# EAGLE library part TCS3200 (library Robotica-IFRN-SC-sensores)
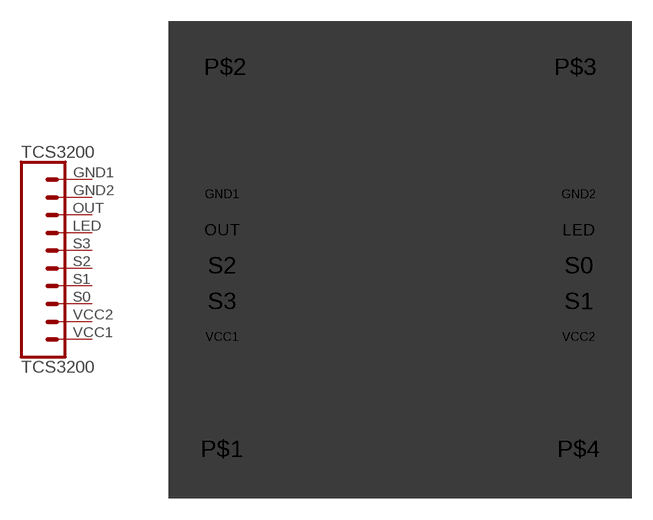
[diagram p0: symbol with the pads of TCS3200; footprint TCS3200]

Designator prefix TCS3200

## TCS3200  [TCS3200]
GND1  GND1  pas
GND2  GND2  pas
LED  LED  pas
OUT  OUT  pas
S0  S0  pas
S1  S1  pas
S2  S2  pas
S3  S3  pas
VCC1  VCC1  pas
VCC2  VCC2  pas

## Footprint TCS3200 (pad centres in mm)
drill 1.118 pad 1.88 long: GND1 -12.69,3.91; GND2 12.71,3.91; LED 12.71,1.37; OUT -12.69,1.37; S0 12.71,-1.17; S1 12.71,-3.71; S2 -12.69,-1.17; S3 -12.69,-3.71; VCC1 -12.69,-6.25; VCC2 12.71,-6.25
drill 2.8: P$1 -12.7,-14.24; P$2 -12.47,12.97; P$3 12.47,12.97; P$4 12.7,-14.24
